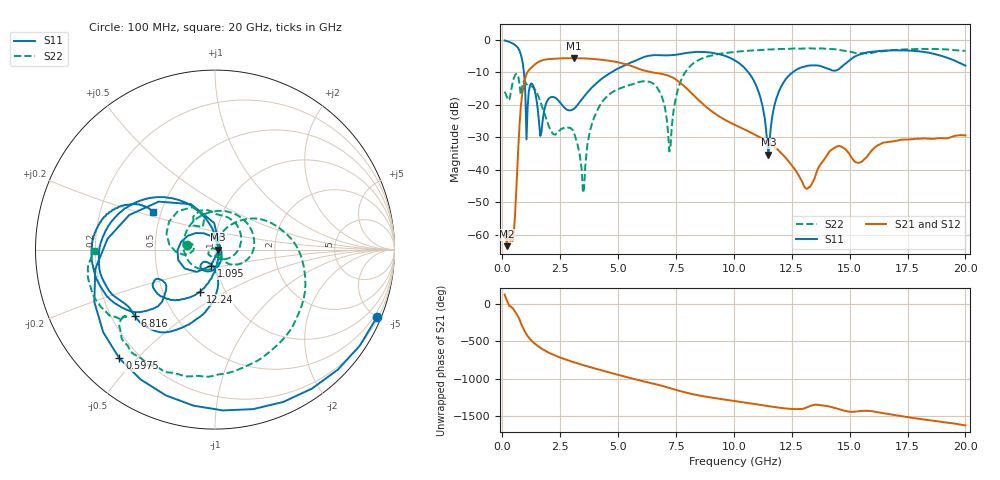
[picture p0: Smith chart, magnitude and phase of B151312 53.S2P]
!  2-Port S-parameters saved by WinCal
! VAR MeasName=S-Parameters (CALIBRATED_DATA) read from VNA (N5244A)
! VAR MeasDate=12/8/2015 5:47:56 PM
! VAR NAME=B151312 53
! VAR FILENAME=B151312 53.S2P
! VAR DATE=12/8/2015 5:47:56 PM
! VAR PHYS_PORTS=1,2
# Hz S DB R 50
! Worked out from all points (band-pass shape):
!   401 points, 100 MHz to 20 GHz, reference 50 ohm
!   highest |S21| = -5.63 dB at 3.085 GHz (marker M1); lowest = -63.5 dB at 199.5 MHz (marker M2)
!   |S21| within 3 dB of the highest: 1.244 GHz to 5.786 GHz (4.542 GHz wide, 129 % of centre)
!   lowest |S11| = -35.4 dB at 11.49 GHz (marker M3), VSWR 1.03, Z = 51.7 + j0.0382 ohm
!   |S11| at or under -10 dB: 932.3 MHz to 4.707 GHz (3.775 GHz wide, 134 % of centre); 10.63 GHz to 12.54 GHz (1.908 GHz wide, 16.5 % of centre)
!   |S22| runs from -47.1 to -2.6 dB; largest |S21 - S12| = 0.002
!   S11 on the Smith chart (normalised r, x): 100 MHz: 0.29, -4.99; 597.5 MHz: 0.13, -0.45; 1.095 GHz: 0.94, -0.17; 6.816 GHz: 0.30, -0.33; 12.24 GHz: 0.76, -0.38; 20 GHz: 0.45, +0.23
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1e8  -0.19 -22.6  -60.79 121.1  -59.83 120.3  -15.96 170.5
1.995e8  -0.38 -44.4  -63.47 39.2  -63.63 39.0  -17.67 166.4
4.4825e8  -1.13 -97.9  -61.86 -60.7  -62.37 -58.5  -13.16 -177.0
5.975e8  -1.86 -131.3  -47.08 -128.7  -47.01 -129.8  -10.46 148.6
8.4625e8  -5.76 158.1  -17.51 69.3  -17.51 69.2  -14.94 131.5
1.095e9  -20.66 -104.3  -9.84 -72.4  -9.84 -72.4  -14.10 87.3
1.44325e9  -17.02 139.0  -7.38 176.7  -7.38 176.7  -15.65 28.2
1.891e9  -19.57 -87.1  -6.04 85.2  -6.04 85.2  -24.24 -58.4
3.085e9  -21.29 -102.6  -5.63 -60.7  -5.63 -60.7  -28.60 -159.3
3.43325e9  -18.29 -87.4  -5.69 -93.9  -5.68 -93.9  -40.21 137.2
4.42825e9  -11.28 -90.6  -6.25 179.2  -6.24 179.2  -18.14 -114.0
5.3735e9  -7.56 -106.9  -7.61 100.7  -7.58 100.6  -14.19 134.0
6.7665e9  -4.71 -139.4  -10.32 -4.1  -10.32 -4.3  -15.59 -27.7
6.81625e9  -4.73 -140.4  -10.37 -8.2  -10.37 -8.4  -16.30 -32.4
7.21425e9  -4.76 -146.7  -11.16 -43.0  -11.13 -43.3  -34.35 -14.2
7.9605e9  -4.02 -157.6  -14.93 -108.1  -14.93 -108.4  -9.39 27.0
1.005e10  -6.34 144.3  -26.21 142.2  -26.22 142.0  -3.71 -64.6
1.149275e10  -35.36 1.2  -31.54 74.5  -31.55 74.4  -2.98 -94.1
1.2239e10  -12.07 -109.6  -36.30 43.0  -36.29 42.8  -2.81 -106.2
1.338325e10  -7.85 -144.4  -44.10 84.2  -44.06 83.5  -2.68 -122.9
1.67165e10  -3.29 -170.9  -31.40 -35.1  -31.33 -35.8  -3.23 -147.5
2e10  -7.93 148.6  -29.43 176.4  -29.53 176.2  -3.41 -179.4
